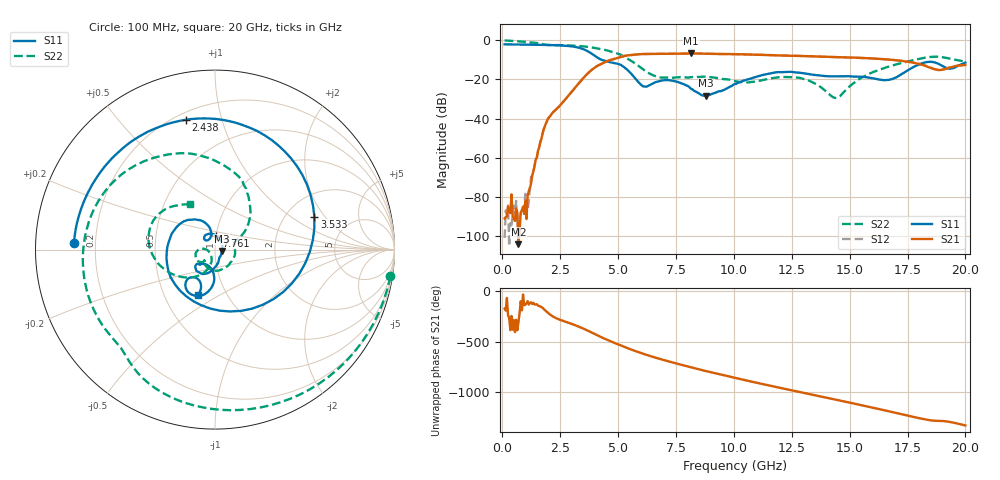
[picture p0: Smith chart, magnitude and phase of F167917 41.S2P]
!  2-Port S-parameters saved by WinCal
! VAR MeasName=S-Parameters (CALIBRATED_DATA) read from VNA (N5242A)
! VAR MeasDate=2016-11-22 9:01:48
! VAR NAME=F167917 41
! VAR FILENAME=F167917 41.S2P
! VAR DATE=2016-11-22 9:01:48
! VAR PHYS_PORTS=1,2
# Hz S DB R 50
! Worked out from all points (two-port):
!   401 points, 100 MHz to 20 GHz, reference 50 ohm
!   highest |S21| = -6.71 dB at 8.159 GHz (marker M1); lowest = -104.0 dB at 697 MHz (marker M2)
!   |S21| within 3 dB of the highest: 4.773 GHz to 16.51 GHz (11.74 GHz wide, 110 % of centre)
!   lowest |S11| = -28.3 dB at 8.806 GHz (marker M3), VSWR 1.08, Z = 53.9 - j0.77 ohm
!   |S11| at or under -10 dB: 4.3 GHz to end of sweep
!   |S22| runs from -29.4 to -0.1 dB; largest |S21 - S12| = 0.005
!   S11 on the Smith chart (normalised r, x): 100 MHz: 0.12, +0.02; 2.438 GHz: 0.24, +0.77; 3.533 GHz: 2.83, +1.58; 7.761 GHz: 1.00, +0.16; 20 GHz: 0.73, -0.40
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1e8  -2.09 177.3  -90.85 -171.0  -100.84 118.8  -0.10 -8.7
6.97e8  -2.17 161.4  -104.04 51.2  -97.26 -177.3  -0.53 -55.9
1.095e9  -2.24 150.5  -79.30 -97.6  -86.44 -74.3  -0.92 -84.3
1.84125e9  -2.37 127.1  -43.75 174.6  -43.72 175.1  -2.21 -129.5
2.43825e9  -2.60 102.7  -33.97 82.1  -33.98 81.8  -2.46 -155.5
3.43325e9  -4.24 30.0  -20.17 -3.5  -20.18 -3.4  -3.05 157.8
3.53275e9  -4.68 18.3  -18.85 -13.7  -18.86 -13.4  -3.16 153.0
4.03025e9  -8.21 -57.8  -13.64 -69.1  -13.59 -68.9  -3.99 128.8
4.5775e9  -10.90 -156.2  -10.42 -127.2  -10.36 -127.5  -5.35 101.3
5.42325e9  -15.32 113.1  -7.71 153.5  -7.71 153.3  -9.46 55.6
6.11975e9  -23.58 119.0  -7.01 96.2  -7.01 96.0  -15.18 28.8
6.7665e9  -20.89 132.1  -6.87 49.9  -6.88 49.7  -18.88 20.5
7.7615e9  -22.07 85.1  -6.82 -12.9  -6.83 -13.0  -18.91 -24.5
8.1595e9  -24.81 54.7  -6.71 -36.6  -6.73 -36.7  -18.83 -48.6
8.80625e9  -28.32 -10.7  -6.88 -74.4  -6.88 -74.4  -18.57 -88.7
1.005e10  -22.32 -78.6  -7.09 -141.6  -7.10 -141.5  -20.86 -132.6
1.19405e10  -16.27 -120.4  -7.76 122.1  -7.70 122.0  -18.81 -146.6
1.338325e10  -17.52 -141.6  -8.19 51.1  -8.15 51.2  -21.33 178.5
1.4428e10  -18.41 -137.0  -8.58 0.1  -8.53 0.1  -29.37 -142.4
1.67165e10  -20.17 -110.6  -9.84 -115.4  -9.88 -115.3  -13.31 -133.8
1.825875e10  -11.28 -109.1  -12.98 164.7  -12.89 164.6  -8.89 -179.6
2e10  -11.39 -110.6  -12.61 104.6  -12.49 104.3  -10.85 118.5
